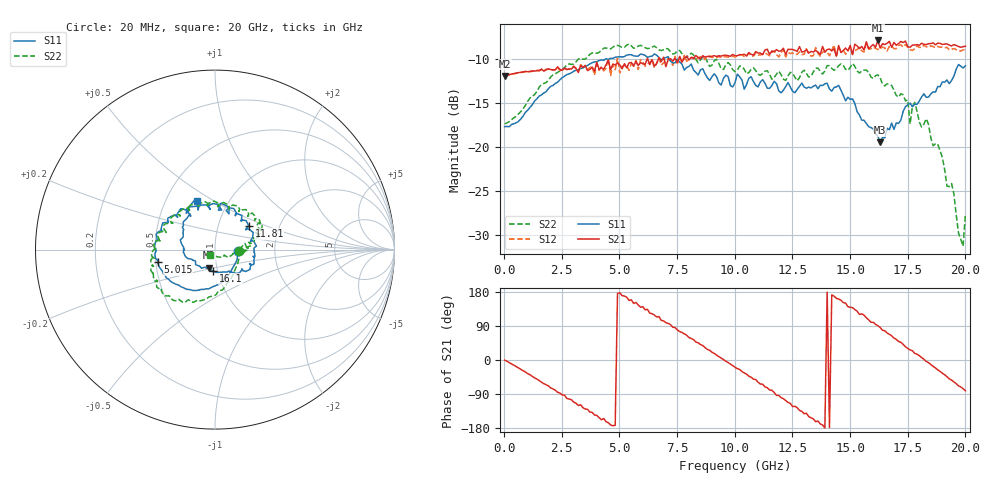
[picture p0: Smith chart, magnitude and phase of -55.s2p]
!Agilent Technologies,N5230A,US43500223,A.07.50.48
!Agilent N5230A: A.07.50.48
!Date: Tuesday, September 15, 2015 18:36:37
!Correction: S11(Full 2 Port(1,2))
!S21(Full 2 Port(1,2))
!S12(Full 2 Port(1,2))
!S22(Full 2 Port(1,2))
!S2P File: Measurements: S11, S21, S12, S22:
# Hz S  RI  R 50
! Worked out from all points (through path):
!   201 points, 20 MHz to 20 GHz, reference 50 ohm
!   highest |S21| = -7.86 dB at 16.2 GHz (marker M1); lowest = -11.9 dB at 20 MHz (marker M2)
!   group delay of S21, straight-line fit = 111 ps
!   lowest |S11| = -19.4 dB at 16.3 GHz (marker M3), VSWR 1.24, Z = 45.6 - j9.26 ohm
!   |S11| at or under -10 dB: start of sweep to 4.381 GHz; 4.497 GHz to 4.526 GHz (28.71 MHz wide, 0.636 % of centre); 7.169 GHz to end of sweep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
!   |S22| runs from -31.3 to -8.3 dB; largest |S21 - S12| = 0.056
!   S11 on the Smith chart (normalised r, x): 20 MHz: 1.30, -0.01; 5.015 GHz: 0.51, -0.08; 11.81 GHz: 1.40, +0.39; 16.1 GHz: 0.96, -0.23; 20 GHz: 0.71, +0.42
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2e7  0.1306 -0.00535  0.2543 -0.00171  0.2537 -0.00239  0.1356 -0.00562
1.8182e9  -0.0116 -0.2064  0.115 -0.25  0.1124 -0.254  0.0184 -0.232
3.4166e9  -0.1994 -0.1993  -0.1666 -0.2305  -0.1812 -0.2196  -0.1411 -0.2831
5.015e9  -0.3192 -0.0709  -0.2933 0.014  -0.2638 0.0149  -0.2998 -0.2271
6.7133e9  -0.3059 0.1042  -0.1342 0.2944  -0.1212 0.2984  -0.3473 -0.0865
7.9121e9  -0.2145 0.186  0.1361 0.3003  0.1427 0.2736  -0.3249 1.64e-05
8.9111e9  -0.0938 0.2204  0.2949 0.1409  0.3036 0.1304  -0.2718 0.0948
1.001e10  0.0229 0.2318  0.3132 -0.1086  0.3052 -0.1157  -0.194 0.1861
1.18082e10  0.1885 0.1318  -0.0217 -0.3583  -0.0294 -0.3354  -0.0344 0.2581
1.34066e10  0.221 -0.0209  -0.3162 -0.1449  -0.2959 -0.1505  0.1514 0.2215
1.43057e10  0.2016 -0.084  -0.3552 0.0718  -0.3699 0.0907  0.2204 0.1623
1.61039e10  -0.00846 -0.119  -0.0265 0.3688  0.00618 0.3644  0.2369 0.0943
1.62038e10  -0.0247 -0.1126  -0.00484 0.4047  0.0267 0.3589  0.2454 0.079
1.63037e10  -0.036 -0.1003  0.0268 0.3656  0.0497 0.358  0.2389 0.0665
1.67033e10  -0.0856 -0.0919  0.1505 0.3707  0.1542 0.3408  0.2194 0.0616
1.75025e10  -0.1727 -0.0205  0.3215 0.1875  0.3296 0.1681  0.1853 -0.0058
1.76024e10  -0.1773 -0.0143  0.3315 0.1658  0.3295 0.1404  0.1353 0.00119
1.78022e10  -0.1753 0.00158  0.3638 0.1146  0.3452 0.113  0.1796 0.00293
1.82018e10  -0.1931 0.0555  0.3844 0.0127  0.3801 -0.00761  0.1354 0.00263
1.94006e10  -0.1378 0.1961  0.2268 -0.3009  0.2003 -0.2995  0.0477 -0.0396
1.99001e10  -0.0987 0.2641  0.0921 -0.3617  0.0674 -0.3515  -0.0119 -0.0245
2e10  -0.1001 0.2729  0.0579 -0.3705  0.0256 -0.3571  -0.0274 -0.0309
